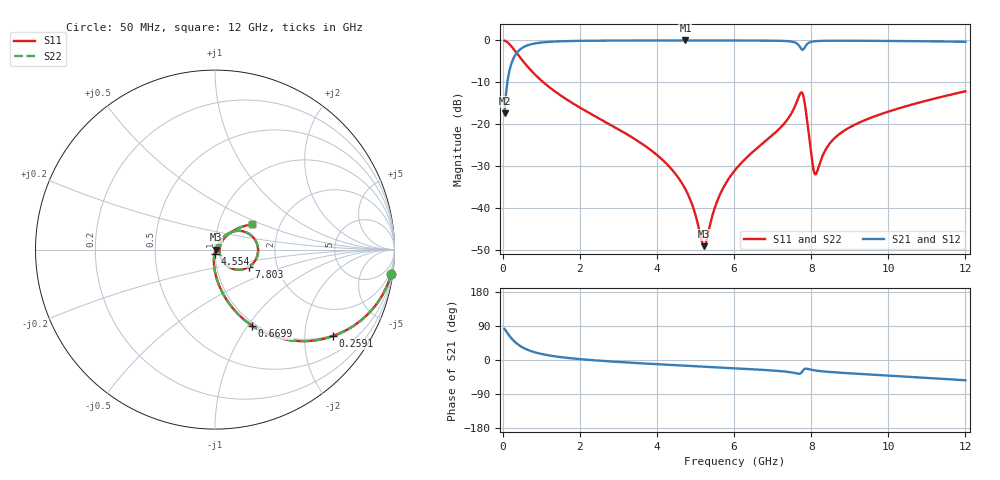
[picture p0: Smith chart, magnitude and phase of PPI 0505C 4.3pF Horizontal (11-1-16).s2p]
# MHz S MA R 50
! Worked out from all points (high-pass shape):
!   1601 points, 50 MHz to 12 GHz, reference 50 ohm
!   highest |S21| = -0.03 dB at 4.74 GHz (marker M1); lowest = -17.3 dB at 50 MHz (marker M2)
!   |S21| within 3 dB of the highest: 361.8 MHz to end of sweep
!   lowest |S11| = -49.0 dB at 5.226 GHz (marker M3), VSWR 1.01, Z = 50.3 - j0.105 ohm
!   |S11| at or under -10 dB: 1.057 GHz to end of sweep
!   |S22| runs from -49.0 to -0.1 dB; largest |S21 - S12| = 0
!   S11 on the Smith chart (normalised r, x): 50 MHz: 1, -14; 259.1 MHz: 0.96, -2.75; 669.9 MHz: 0.96, -1.05; 4.554 GHz: 0.99, -0.05; 7.803 GHz: 1.44, -0.29; 12 GHz: 1.43, +0.43
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50  0.9907 -8.0  0.1359 82.0  0.1359 82.0  0.9907 -8.0
154.5625  0.9205 -23.5  0.3905 66.5  0.3905 66.5  0.9205 -23.5
259.125  0.8143 -36.3  0.5799 53.6  0.5799 53.6  0.8143 -36.3
669.9062  0.4729 -63.9  0.88 25.9  0.88 25.9  0.4729 -63.9
1155.375  0.2901 -76.8  0.9554 12.9  0.9554 12.9  0.2901 -76.8
2044.156  0.1544 -87.3  0.9858 1.9  0.9858 1.9  0.1544 -87.3
4038.312  0.04184 -97.2  0.9959 -11.3  0.9959 -11.3  0.04184 -97.2
4553.656  0.02325 -96.2  0.9962 -14.1  0.9962 -14.1  0.02325 -96.2
4740.375  0.01686 -93.8  0.9963 -15.1  0.9963 -15.1  0.01686 -93.8
5225.844  0.003557 -17.0  0.9961 -17.6  0.9961 -17.6  0.003557 -17.0
5599.281  0.01344 53.9  0.9958 -19.6  0.9958 -19.6  0.01344 53.9
6025  0.02852 59.7  0.995 -21.9  0.995 -21.9  0.02852 59.7
7242.406  0.0954 53.9  0.9844 -29.7  0.9844 -29.7  0.0954 53.9
7593.438  0.1696 38.1  0.9361 -34.7  0.9361 -34.7  0.1696 38.1
7727.875  0.2368 7.1  0.8111 -34.9  0.8111 -34.9  0.2368 7.1
7802.562  0.2131 -26.5  0.7864 -25.9  0.7864 -25.9  0.2131 -26.5
8019.156  0.03864 -44.8  0.9628 -26.0  0.9628 -26.0  0.03864 -44.8
8131.188  0.02599 7.8  0.9783 -28.0  0.9783 -28.0  0.02599 7.8
8385.125  0.05091 46.9  0.9873 -30.8  0.9873 -30.8  0.05091 46.9
8683.875  0.07366 50.8  0.9889 -33.1  0.9889 -33.1  0.07366 50.8
10013.31  0.1424 46.2  0.9828 -41.2  0.9828 -41.2  0.1424 46.2
12000  0.2476 34.7  0.9605 -53.5  0.9605 -53.5  0.2476 34.7
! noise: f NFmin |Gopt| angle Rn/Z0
50  0.0005549  0.9143  2.083  0.001426
1372  0.00492  0.728  5.401  0.003591
2701  0.008087  0.6832  9.615  0.004913
4031  0.01102  0.6595  13.85  0.006098
5360  0.01409  0.6502  18.04  0.007475
6682  0.01905  0.6753  22.16  0.01092
8012  0.05528  0.853  26.73  0.07598
9341  0.02458  0.6589  30.39  0.01286
1.067e+04  0.02675  0.6489  34.13  0.01327
1.2e+04  0.03034  0.6557  37.84  0.01511
